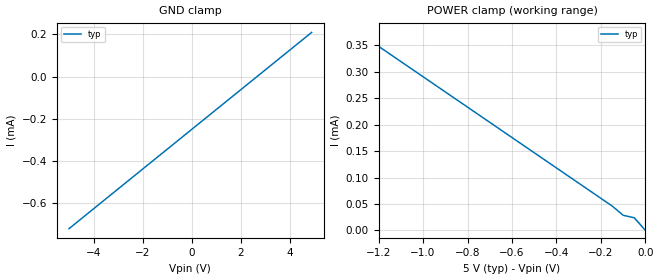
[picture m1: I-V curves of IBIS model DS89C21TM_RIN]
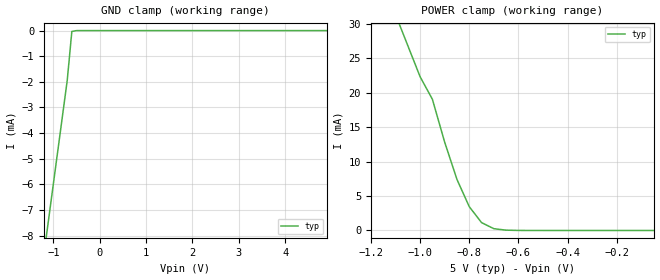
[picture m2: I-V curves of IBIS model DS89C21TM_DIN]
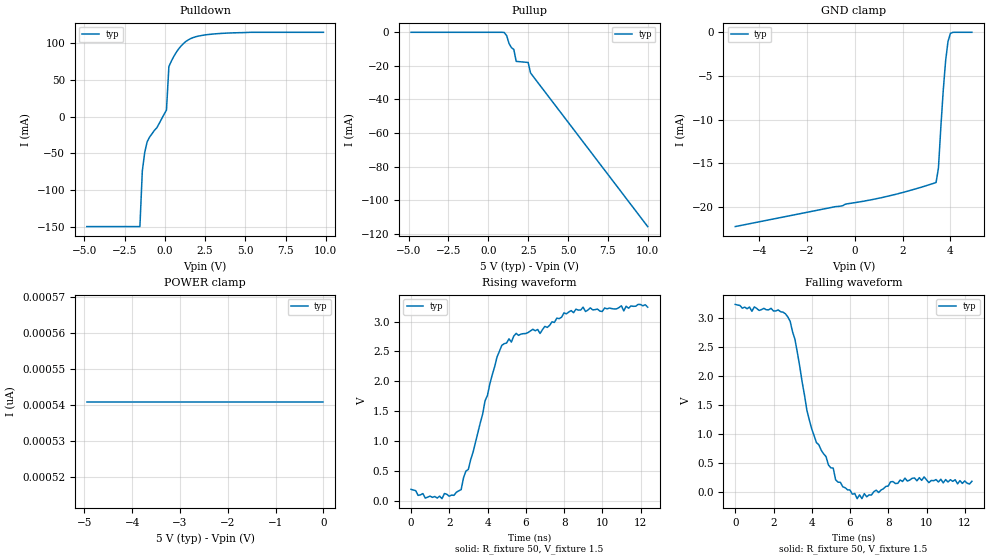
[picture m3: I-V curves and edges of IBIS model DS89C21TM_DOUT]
|   National Semiconductor Corporation
|   IBIS Model of DS89C21TM
|   Differential CMOS Line Driver and Receiver Pair
|   8 Lead SOIC Package
[IBIS Ver]   3.2
[Comment Char]   |_char
[File name]   ds89c21tm.ibs
[File Rev]   1.0
[Date]   06/05/03
[Source]
Empirical Data, Typ Only;
[Notes]
Created by Davor Glisic
[Disclaimer]
(C) Copyright National Semiconductor Corporation 2002
   All rights reserved
   National Semiconductor Corporation hereby grants
the user of this IBIS model a non-exclusive, nontransferable
license to use this IBIS model under the following terms.
Before using this IBIS model, the user should read this
license.  If the user does not accept these terms,  the
IBIS model should be returned to National within 30 days.
   The user is granted this license only to use the
IBIS model and is not granted rights to sell, load, rent,
lease or license the IBIS model in whole or in part, or in
modified form to anyone other than user. User may modify
the IBIS model to suit its specific applications but rights
to derivative works and such modifications shall belong to
National.
   This IBIS model is provided on an "AS IS" basis and
National makes absolutely no warranty with respect to the
information contained herein.NATIONAL DISCLAIMS AND CUSTOMER
WAIVES ALL WARRANTIES, EXPRESS OR IMPLIED, INCLUDING
WARRANTIES OF MERCHANTABILITY OR FITNESS FOR A PARTICULAR
PURPOSE. The entire risk as to quality and performance is
with the Customer. ACCORDINGLY, IN NO EVENT SHALL THE
COMPANY BE LIABLE FOR ANY DAMAGES, WHETHER IN CONTRACT OR
TORT,INCLUDING ANY LOST PROFITS OR OTHER INCIDENTAL,
CONSEQUENTIAL, EXEMPLARY, OR PUNITIVE DAMAGES ARISING OUT
OF THE USE OR APPLICATION OF THE IBIS model provided in
this package.Further, National reserves the right to make
changes without notice to any product herein to improve
reliability, function, or design. National does not convey
any license under patent rights or any other intellectual
property rights, including those of third parties.
   National is not obligated to provide maintenance or support
for the licensed IBIS model.
Contact National at ATTN:INTERFACE APPLICATIONS/IBIS MODELS.
5 Foden Road, M/S 03-03, South Porltand, ME 04106
(207) 541-6031
[Copyright]
(c) Copyright 2002 National Semiconductor Corp.
[Component]   DS89C21TM
Si_location Pin
Timing_location Pin
[Manufacturer]   National Semiconductor Corp.
[Package]
|   TYP   MIN   MAX
R_pkg   50.0m   50.0m   50.0m
L_pkg   1.164nH   1.04n   1.33n
C_pkg   0.207pF   0.178p   0.245p
[Pin]   signal_name   model_name   R_pin   L_pin   C_pin
1   VDD   POWER   50.0m   1.33n   0.245p
2   ROUT   DS89C21TM_ROUT   50.0m   1.04n   0.178p
3   DIN   DS89C21TM_DIN   50.0m   1.04n   0.178p
4   GND   GND   50.0m   1.33n   0.245p
5   DOUT-   DS89C21TM_DOUT   50.0m   1.33n   0.245p
6   DOUT+   DS89C21TM_DOUT   50.0m   1.04n   0.178p
7   RIN-   DS89C21TM_RIN   50.0m   1.04n   0.178p
8   RIN+   DS89C21TM_RIN   50.0m   1.33n   0.245p
[Diff Pin] inv_pin   vdiff   tdelay_typ   tdelay_min   tdelay_max
| The '+' pin is Diff_pin and the '-' pin is the inv_pin
| Receiver Vth = +/-100mV
6   5   0   0   0   0
8   7   0.1   0   0   0
| Models and submodels in the file (4): DS89C21TM_RIN (Input), DS89C21TM_DIN (Input), DS89C21TM_DOUT (Output), DS89C21TM_ROUT (Output)
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|   Receiver Input  MODEL
[Model]   DS89C21TM_RIN
Model_type   Input
|Signals   RIN+,RIN-
Vinh = 2.0
Vinl = 0.8
|   typ   min   max
C_comp   1.0pF   NA   NA
|   typ   min   max
[Temperature Range]   25.0   NA   NA
[Voltage range]   5.0V   4.5V   5.5V
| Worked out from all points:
|   POWER clamp passes 1 mA (typ) near -3.47 V on its own axis
[Power_clamp]
| Note that the[POWER_clamp]voltage table is referenced to Vcc
| and is calculated using Vtable=Vcc - Vmeasured.
|   Voltage   I(typ)   I(min)   I(max)
-4.95V    1.424mA    NA         NA
-1.3V     376.4uA    NA         NA
-150mV    46.26uA    NA         NA
-100mV    28.71uA    NA         NA
-50mV     23.94uA    NA         NA
0V        0A         NA         NA
[GND_clamp]
|   Voltage   I(typ)   I(min)   I(max)
-5V       -722.5uA   NA         NA
-3.6V     -590.4uA   NA         NA
-2.9V     -524.7uA   NA         NA
4.9V      209.6uA    NA         NA
|   Driver Input  MODEL
[Model]   DS89C21TM_DIN
Model_type   Input
|Signals   DIN
Vinh = 2.0
Vinl = 0.8
|   typ   min   max
C_comp   1.0pF   NA   NA
|   typ   min   max
[Temperature Range]   25.0   NA   NA
[Voltage range]   5.0V   4.5V   5.5V
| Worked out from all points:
|   GND clamp passes 1 mA (typ) near -0.65 V on its own axis
|   POWER clamp passes 1 mA (typ) near -0.74 V on its own axis
[Power_clamp]
| Note that the[POWER_clamp]voltage table is referenced to Vcc
| and is calculated using Vtable=Vcc - Vmeasured.
|   Voltage   I(typ)   I(min)   I(max)
-5V       384mA      NA         NA
-1.1V     31.38mA    NA         NA
-1.05V    26.86mA    NA         NA
-1V       22.34mA    NA         NA
-950mV    19.06mA    NA         NA
-900mV    12.82mA    NA         NA
-850mV    7.406mA    NA         NA
-800mV    3.451mA    NA         NA
-750mV    1.14mA     NA         NA
-700mV    256.9uA    NA         NA
-650mV    46.9uA     NA         NA
-50mV     212pA      NA         NA
[GND_clamp]
|   Voltage   I(typ)   I(min)   I(max)
-5V       -60mA      NA         NA
-1.2V     -8.7mA     NA         NA
-1.1V     -7.35mA    NA         NA
-700mV    -1.95mA    NA         NA
-600mV    -33.2uA    NA         NA
-400mV    -21.5nA    NA         NA
4.9V      3.04pA     NA         NA
|   Driver Output  MODEL
[Model]   DS89C21TM_DOUT
Model_type   Output
| Signals   DOUT+,DOUT-
Vmeas = 1.5V   |Reference voltage for timing measurements
Cref = 50pF   |Timing specification test load capacitance value
Rref = 50   |Note: 100 Ohm between the two driver outputs
Vref = 1.5V   |Timing specification test load voltage; GND
| variable   typ   min   max
C_comp   3.0pF   NA   NA
|   typ   min   max
[Temperature Range]   25.0   NA   NA
[Voltage range]   5.0V   4.5V   5.5V
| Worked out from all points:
|   slope of the pulldown table from 0 to 0.75 V, typ, clamps not added: 8.93 ohm
|   falling waveform, R_fixture 50, V_fixture 1.5: 20-80 % time 1.27ns typ, NA min, NA max; typ from 3.24 V to 0.19 V
|   rising waveform, R_fixture 50, V_fixture 1.5: 20-80 % time 1.65ns typ, NA min, NA max; typ from 0.192 V to 3.24 V
[Pulldown]
|   Voltage   I(typ)   I(min)   I(max)
-4.85V    -150.1mA   NA         NA
-1.55V    -150.1mA   NA         NA
-1.4V     -74.09mA   NA         NA
-1.25V    -48.72mA   NA         NA
-1.1V     -34.41mA   NA         NA
100mV     8.913mA    NA         NA
250mV     68.22mA    NA         NA
700mV     87.35mA    NA         NA
1.3V      102.4mA    NA         NA
2.05V     109.6mA    NA         NA
3.55V     113.5mA    NA         NA
9.85V     114.9mA    NA         NA
[Pullup]
|   Voltage   I(typ)   I(min)   I(max)
| Note that the[Pullup]voltage table is referenced to Vcc
| and is calculated using Vtable=Vcc - Vmeasured.
-4.85V    379pA      NA         NA
1V        -133.6uA   NA         NA
1.15V     -1.985mA   NA         NA
1.3V      -6.657mA   NA         NA
1.45V     -9.148mA   NA         NA
1.6V      -10.2mA    NA         NA
1.75V     -17.34mA   NA         NA
2.5V      -17.99mA   NA         NA
2.65V     -24.2mA    NA         NA
10V       -115.8mA   NA         NA
[GND_clamp]
|   Voltage   I(typ)   I(min)   I(max)
-5V       -22.25mA   NA         NA
1.1V      -18.95mA   NA         NA
2V        -18.35mA   NA         NA
3.4V      -17.2mA    NA         NA
3.5V      -15.54mA   NA         NA
3.6V      -10.88mA   NA         NA
3.7V      -6.672mA   NA         NA
3.8V      -3.257mA   NA         NA
3.9V      -1.038mA   NA         NA
4V        -130.2uA   NA         NA
4.1V      -5.17uA    NA         NA
4.9V      391pA      NA         NA
[POWER_clamp]
|   Voltage   I(typ)   I(min)   I(max)
| Note that the[POWER_clamp]voltage table is referenced to Vcc
| and is calculated using Vtable=Vcc - Vmeasured.
-4.95V    541pA      NA         NA
-4.9V     541pA      NA         NA
-4.85V    541pA      NA         NA
0V        541pA      NA         NA
[Ramp]
|   typ   min   max
dV/dt_r   2.52/2.2n   NA   NA
dV/dt_f   2.52/2.1n   NA   NA
R_load = 100Ohm
[Falling Waveform]
R_fixture=50
V_fixture=1.5
|Time   V(typ)   V(min)   V(max)
0s        3.24V      NA         NA
2.745ns   3.025V     NA         NA
3.12ns    2.636V     NA         NA
3.745ns   1.413V     NA         NA
4.245ns   856.7mV    NA         NA
5.12ns    417.5mV    NA         NA
5.245ns   217mV      NA         NA
6.37ns    -109.6mV   NA         NA
8.87ns    244.4mV    NA         NA
12.37ns   190mV      NA         NA
[Rising Waveform]
R_fixture=50
V_fixture=1.5
|Time   V(typ)   V(min)   V(max)
0s        191.6mV    NA         NA
1.62ns    35.83mV    NA         NA
2.62ns    187.4mV    NA         NA
3.245ns   816mV      NA         NA
4.495ns   2.406V     NA         NA
5.12ns    2.71V      NA         NA
6.745ns   2.8V       NA         NA
7.995ns   3.145V     NA         NA
8.995ns   3.24V      NA         NA
12.37ns   3.24V      NA         NA
